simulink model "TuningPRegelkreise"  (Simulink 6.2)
settings: Solver=ode3  StartTime=0.0  StopTime=8  MaxStep=.01  RelTol=1e-3  SampleTimeConstraint=Specified
libraries: simulink_extras x4

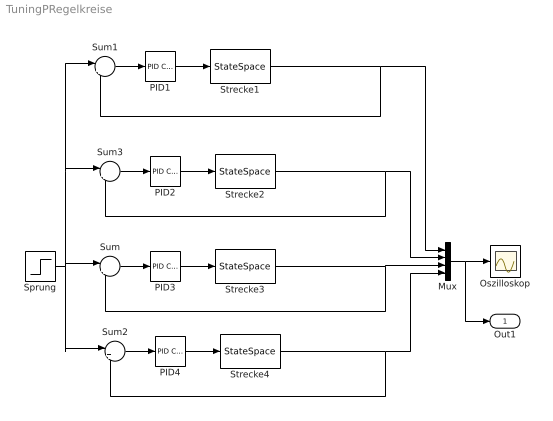
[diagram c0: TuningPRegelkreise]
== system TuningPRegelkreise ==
  Mux : Mux
  Oszilloskop : Scope
  PID1 : simulink_extras/Additional Linear/PID Controller  P=50  I=0  D=0
  PID2 : simulink_extras/Additional Linear/PID Controller  P=100  I=0  D=0
  PID3 : simulink_extras/Additional Linear/PID Controller  P=145  I=0  D=0
  PID4 : simulink_extras/Additional Linear/PID Controller  P=180  I=0  D=0
  Sprung : Step  Time=0  SampleTime=0
  Strecke{1..4} (4 alike) : StateSpace  A=[-0.404 0.229;0.179 -0.554];  B=[1.189 ;-0.037]  C=[0 0.175]  D=0
  Sum{,1..3} (4 alike) : Sum  Inputs=|+-
  Out1 : Outport
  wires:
  PID3/1 -> Strecke3/1
  Sprung/1 -> Sum/1, Sum2/1, Sum1/1, Sum3/1
  Sum/1 -> PID3/1
  Strecke3/1 -> Sum/2, Mux/3
  PID1/1 -> Strecke1/1
  Sum1/1 -> PID1/1
  Strecke1/1 -> Sum1/2, Mux/1
  PID4/1 -> Strecke4/1
  Sum2/1 -> PID4/1
  Strecke4/1 -> Sum2/2, Mux/4
  Mux/1 -> Oszilloskop/1, Out1/1
  PID2/1 -> Strecke2/1
  Sum3/1 -> PID2/1
  Strecke2/1 -> Sum3/2, Mux/2
